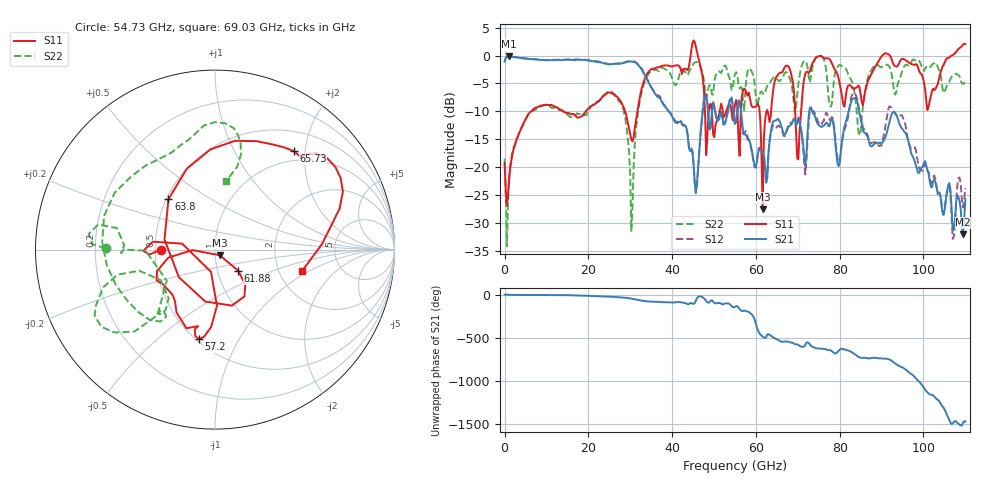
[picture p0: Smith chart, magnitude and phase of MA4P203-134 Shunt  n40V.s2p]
!Keysight Technologies,N5247B,US61255204,A.15.70.20
!Date: Friday, October 21, 2022 15:19:09
!Correction: S11(C  4-Port  )
!S31(C  4-Port  )
!S13(C  4-Port  )
!S33(C  4-Port  )
!S2P File: Measurements: S11, S31, S13, S33:
# Hz S  dB  R 50
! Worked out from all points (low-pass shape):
!   401 points, 10 MHz to 110 GHz, reference 50 ohm
!   highest |S21| = -0.15 dB at 1.11 GHz (marker M1); lowest = -32.1 dB at 109.5 GHz (marker M2)
!   |S21| within 3 dB of the highest: start of sweep to 33.21 GHz
!   lowest |S11| = -27.6 dB at 61.6 GHz (marker M3), VSWR 1.09, Z = 52.7 - j3.35 ohm
!   |S11| at or under -10 dB: start of sweep to 6.347 GHz; 14.1 GHz to 19.37 GHz (5.273 GHz wide, 31.5 % of centre); 28.78 GHz to 31.71 GHz (2.932 GHz wide, 9.69 % of centre)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
!   |S22| runs from -34.2 to 0.0 dB; largest |S21 - S12| = 0.16
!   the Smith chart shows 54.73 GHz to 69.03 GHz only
!   S11 on the Smith chart (normalised r, x): 54.73 GHz: 0.53, -0.00; 57.2 GHz: 0.52, -0.69; 61.88 GHz: 1.26, -0.31; 63.8 GHz: 0.51, +0.34; 65.73 GHz: 0.82, +1.78; 69.03 GHz: 2.68, -0.86
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1e7  -19.34 1.5  -1.07 -0.2  -1.08 -0.1  -18.48 -1.7
1.1099e9  -21.97 71.7  -0.15 -0.1  -0.13 -0.0  -21.75 103.6
1.843332e10  -10.87 86.5  -0.76 -9.3  -0.71 -9.2  -10.51 72.9
3.025725e10  -15.05 124.2  -1.08 -44.7  -0.98 -44.0  -31.41 37.9
3.685665e10  -2.10 -179.5  -7.55 -81.7  -7.14 -80.3  -2.76 -172.4
4.538088e10  2.42 94.0  -22.71 -96.8  -22.70 -97.1  -1.26 146.2
4.813062e10  -17.84 61.0  -7.20 -71.7  -6.98 -72.5  -7.59 119.8
5.473002e10  -10.36 -179.8  -10.98 -147.2  -11.10 -149.4  -4.32 179.4
5.5005e10  -8.73 -175.7  -12.25 -140.6  -12.50 -142.4  -3.29 177.4
5.72048e10  -5.91 -100.3  -14.16 175.7  -14.02 -176.2  -9.90 -147.1
6.16044e10  -27.59 -49.5  -17.43 -125.0  -17.50 -123.2  -6.74 -131.8
6.187938e10  -15.13 -42.3  -17.70 -134.1  -17.83 -132.4  -6.96 -129.0
6.38042e10  -8.36 132.8  -12.61 -122.8  -13.10 -121.7  -4.30 -171.8
6.572902e10  -3.06 51.4  -11.87 -176.6  -12.84 -167.6  -4.56 114.4
6.902872e10  -6.04 -14.0  -11.32 155.3  -11.40 148.9  -8.29 80.9
7.342832e10  -1.46 -175.5  -9.98 116.9  -9.88 112.0  -2.31 158.9
8.085265e10  -8.77 -104.1  -13.87 88.4  -14.28 87.3  -2.03 -129.6
9.185165e10  0.12 89.1  -12.02 -32.2  -9.09 -24.8  -1.99 76.4
9.79011e10  -1.69 174.5  -18.97 124.0  -16.44 121.9  -0.82 -176.3
1.023007e11  -5.92 -69.1  -22.59 -89.7  -21.98 -83.2  -1.45 -114.5
1.0945e11  2.01 39.4  -32.05 -50.2  -27.25 -45.4  -5.06 2.7
1.1e11  2.07 46.2  -25.73 -31.8  -23.73 -30.1  -5.50 12.1
